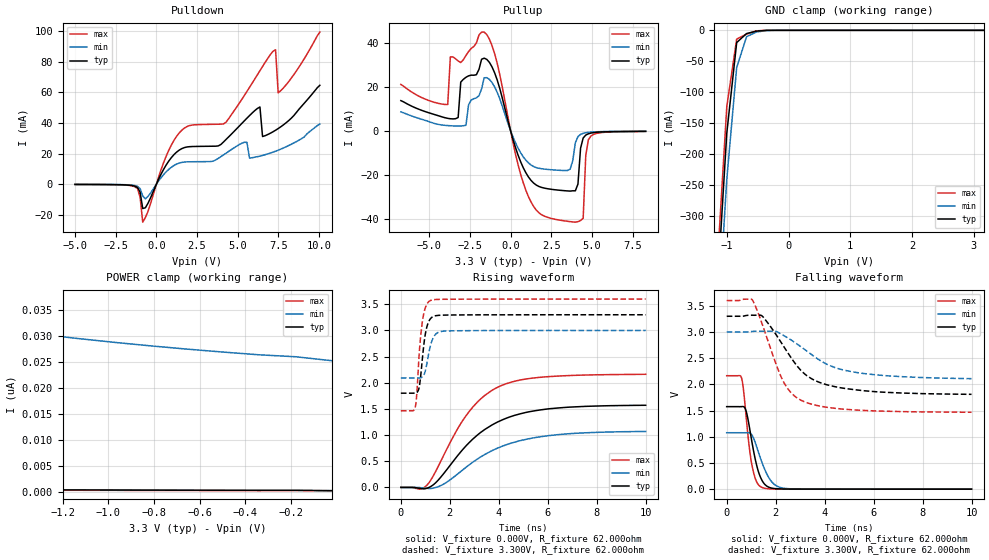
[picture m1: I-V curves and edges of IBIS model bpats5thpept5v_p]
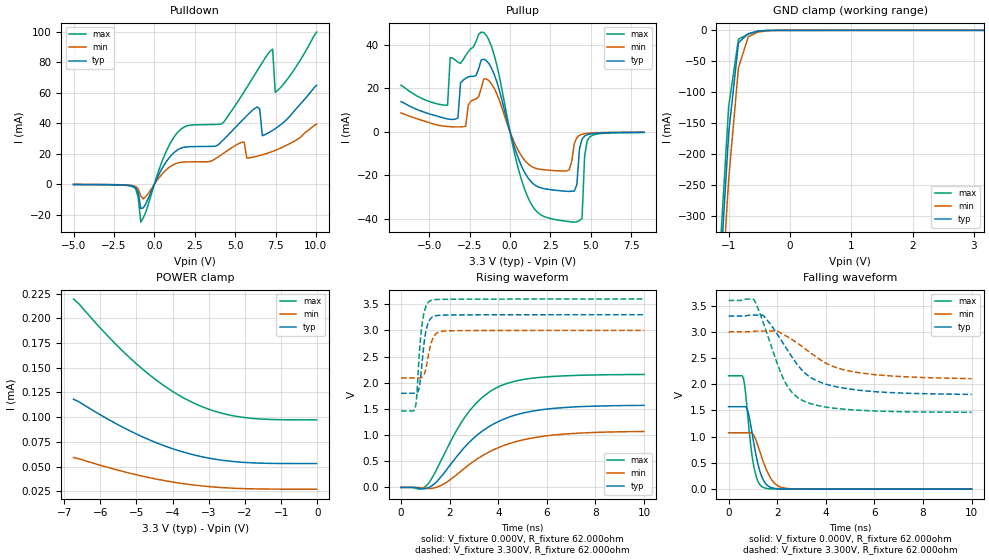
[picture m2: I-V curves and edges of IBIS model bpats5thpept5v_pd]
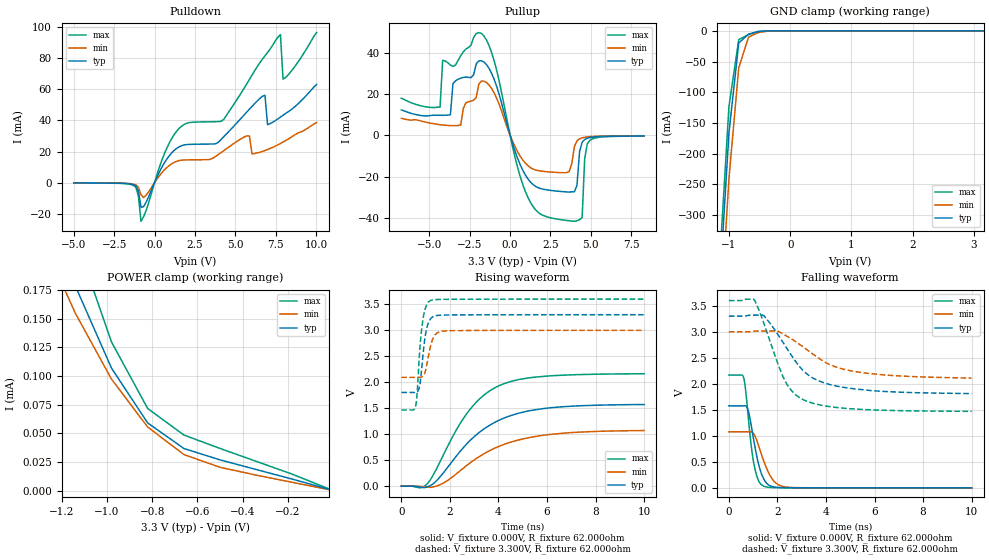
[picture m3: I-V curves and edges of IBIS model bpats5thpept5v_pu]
[IBIS Ver]  4.0
[File Name]  lpc13xx_hvqfn33_rev.ibs
[File Rev]  1.0
[Date]   Fri Oct 15 17:01:21 PDT 2006
[Source]   Package model from Ansoft Q3D Extractor 7.1.1
[Notes]   IO models Rev 0.20 IBIS Model Design Automation Generation
[Copyright] NXP Semiconductors 2006. All rights reserved.
|   LPC134x/LPC131x IBIS Model
[Disclaimer]
| NXP Semiconductors warrants and represents that the IBIS models
| identified herein are owned by NXP Semiconductors (NXP).  The
| models provided are not warranted as fully representing all of the
| operating characteristics and specifications of the semiconductor
| products to which the models relate.  Moreover, unless there is a
| signed, written agreement to the contrary, these models are furnished
| on an "as is" basis without support or warranty of any kind, either
| expressed or implied, regarding the use thereof, and NXP
| specifically disclaims all implied warranties of merchantability and
| fitness of the models for any purpose.
| NXP does not assume any liability arising out of the application
| or use of these IBIS models including infringement of patents and
| copyrights, nor does NXP convey any license under its patents and
| copyrights or the rights of others.
| NXP provides IBIS models as a service to our customers.  You and
| your company shall not distribute, convey, sell, or give these models
| to anyone else without receiving prior written permission from
| NXP.
[Component]   lpc13xx
[Manufacturer]  NXP
[Package]
|   Typ   Min   Max
R_pkg   1.15e-1   0.24e-1   4.46e-1
L_pkg   6.44e-9   5.71e-9   7.17e-9
C_pkg   0.5e-12   0.5e-12   0.5e-12
| (Pin and IO model definitions)
| IMPORTANT NOTES:
| The lpc13xx GPIO pins, excluding the I2C, have programmable input
| configurations. For this reason, three models are supplied for those basic
| padcells. Each model is identified by a unique suffix code at the end of
| the modelname:
| _p=plain input, _pd=pulldown enabled, _pu=pullup enabled
| The model_name for each of the GPIO pins in the [Pin] table below reflects
| the default state of that pin on power up (input with pullup enabled).
| The user may modify the model_name for a specific P#.# pin if that pin's
| input configuration is programmed differently from the default in the
| actual application. However, the model_names for all other pins are
| non-configurable and should not be altered.
| All GPIO padcells have 5ns slew rate control when operated as outputs,
| unless otherwise noted.
|This model covers both the USB version LPC134x and the non usb version
|of the LPC1300. Uncomment the appropriate model for the correct function.
[Pin]   signal_name   model_name   | comments
1   PIO2_0   bpts5ptpht5v_pu
2   PIO0_0   bpts5ptpht5v_pu   | Reset Pad
3   PIO0_1   bpts5ptpht5v_pu
4   XTALIN   NC
5   XTALOUT   NC
6   VDDIO_EXT_1   POWER
7   PIO1_8   bpts5ptpht5v_pu
8   PIO0_2   bpts5ptpht5v_pu
9   PIO0_3   bpts5ptpht5v_pu
10   PIO0_4   iic3m4sdat5v_400k   |iic3m20m4sdat5v_pd
11   PIO0_5   iic3m4sdat5v_400k   |iic3m20m4sdat5v_pd
12   PIO1_9   bpts5ptpht5v_pu
13   USB_DM   usb11f1_iom_hs
14   USB+DP   usb11f1_iop_hs
|13   PIO3_4   bpts5ptpht5v_pu
|14   PIO3_5   bpts5ptpht5v_pu
15   PIO0_6   bpts5ptpht5v_pu
16   PIO0_7   bpts5ptpht5v_pu   |bpt20ms5ptpht5v_pd_v1
17   PIO0_8   bpts5ptpht5v_pu
18   PIO0_9   bpts5ptpht5v_pu
19   PIO0_10   bpts5ptpht5v_pu
20   PIO1_10   bpats5thpept5v_pu
21   PIO0_11   bpats5thpept5v_pu
22   PIO1_0   bpats5thpept5v_pu
23   PIO1_1   bpats5thpept5v_pu
24   PIO1_2   bpats5thpept5v_pu
25   PIO1_3   bpats5thpept5v_pu
26   PIO1_4   bpats5thpept5v_pu   |bpats5thpept5v_pdwu_v1
27   PIO1_11   bpats5thpept5v_pu
28   PIO3_2   bpts5ptpht5v_pu
29   VDDMAIN_EXT   POWER
30   PIO1_5   bpts5ptpht5v_pu
31   PIO1_6   bpts5ptpht5v_pu
32   PIO1_7   bpts5ptpht5v_pu
| Models and submodels in the file (9): bpats5thpept5v_p (I/O), bpats5thpept5v_pd (I/O), bpats5thpept5v_pu (I/O), bpts5ptpht5v_p (I/O), bpts5ptpht5v_pd (I/O), bpts5ptpht5v_pu (I/O), iic3m4sdat5v_400k (I/O_open_drain), usb11f1_iom_hs (I/O), usb11f1_iop_hs (I/O)
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| bpats5thpept5v
|   Bidirectional Pad 3v3
|   CMOS
|   Characterized at Core 1.8V and I/O 3.3V
| Plain input Mode (p1=0, p2=1)
[Model]   bpats5thpept5v_p | of bpats5thpept5v
Model_type   I/O
Polarity   Non-Inverting
Enable   Active-Low
|  Reciever Thresholds
Vinl   = 0.54V
Vinh   = 1.26V
| AC Test Load Conditions
Vref   = 0
Cref   = 1.2e-11
Rref   = 1000000000
Vmeas   = 0.9
| [Process Range]   typical   min   max
| C_comp edge width   400.000ps   400.000ps   400.000ps
| C_comp Tstrobe   40.000fs   40.000fs   40.000fs
C_comp   2.539pF   2.402pF   2.679pF
[Temperature Range]   25   125   -40
[Voltage Range]   3.30V   3.00V   3.60V
[GND Clamp Reference]   0.00V   0.00V   0.00V
[Pulldown Reference]   0.00V   0.00V   0.00V
[POWER Clamp Reference]   3.30V   3.00V   3.60V
[Pullup Reference]   3.30V   3.00V   3.60V
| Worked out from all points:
|   slope of the pulldown table from 0 to 0.495 V, typ, clamps not added: 46.5 ohm
|   slope of the pullup table from 0 to 0.495 V, typ, clamps not added: 41.9 ohm
|   GND clamp passes 1 mA (typ) near -0.48 V on its own axis
|   rising waveform, V_fixture 0.000V, R_fixture 62.000ohm: 20-80 % time 2.15ns typ, 2.37ns min, 1.8ns max; typ from 0 V to 1.57 V
|   falling waveform, V_fixture 0.000V, R_fixture 62.000ohm: 20-80 % time 411ps typ, 539ps min, 319ps max; typ from 1.57 V to 0 V
|   rising waveform, V_fixture 3.300V, R_fixture 62.000ohm: 20-80 % time 225ps typ, 260ps min, 215ps max; typ from 1.8 V to 3.3 V
|   falling waveform, V_fixture 3.300V, R_fixture 62.000ohm: 20-80 % time 1.53ns typ, 1.95ns min, 1.1ns max; typ from 3.3 V to 1.81 V
[GND Clamp]
| ref voltage   0.00V   0.00V   0.00V
|   Voltage   I(typ)   I(min)   I(max)
-5V       -7.933A    -7.953A    -7.929A
-1.16V    -429.6mA   -501mA     -389.4mA
-1V       -166.1mA   -240.8mA   -123.1mA
-840mV    -19.82mA   -60.19mA   -14.18mA
-680mV    -5.225mA   -10.28mA   -6.152mA
-520mV    -1.304mA   -2.7mA     -818.1uA
-200mV    -132.3nA   -9.731uA   -2.769nA
3.16V     216.3pA    26.32nA    148.8pA
[Power Clamp]   | Vtable = Vcc - Vpad
| ref voltage   3.30V   3.00V   3.60V
|   Voltage   I(typ)   I(min)   I(max)
-6.74V    1.379nA    125.5nA    723.8pA
-4.66V    863pA      70.57nA    560.5pA
-2.42V    509.5pA    38.28nA    388.3pA
-2.26V    489.9pA    36.89nA    376pA
-2.1V     470.8pA    35.59nA    363.8pA
-1.78V    434.1pA    33.27nA    339.4pA
-1.62V    416.5pA    32.24nA    327.2pA
-1.3V     382.5pA    30.41nA    302.8pA
-820mV    334.3pA    28.18nA    266.3pA
-340mV    288.9pA    26.43nA    229.9pA
-180mV    281.7pA    26.06nA    265.9pA
-20mV     233pA      25.29nA    176.8pA
[Pulldown]
| ref voltage   0.00V   0.00V   0.00V
|   Voltage   I(typ)   I(min)   I(max)
-5V       -187.5uA   -145.8uA   -211.8uA
-1.32V    -1.32mA    -939.5uA   -1.723mA
-1V       -5.324mA   -2.961mA   -8.618mA
-840mV    -15.95mA   -7.735mA   -24.89mA
1.4V      22.26mA    13.79mA    33.48mA
4.28V     29.27mA    20.27mA    40.55mA
5.56V     43.15mA    27.33mA    60.63mA
6.36V     50.49mA    18.36mA    74.24mA
6.52V     31.16mA    18.79mA    76.97mA
7.32V     35.27mA    21.55mA    87.95mA
7.48V     36.36mA    22.22mA    59.78mA
10.04V    64.68mA    39.32mA    99.49mA
[Pullup]   | Vtable = Vcc - Vpad
| ref voltage   3.30V   3.00V   3.60V
|   Voltage   I(typ)   I(min)   I(max)
-6.74V    13.67mA    8.53mA     21.02mA
-3.86V    5.598mA    2.307mA    11.88mA
-3.7V     5.416mA    2.227mA    33.56mA
-2.74V    24.29mA    2.441mA    34.22mA
-1.62V    32.99mA    24.07mA    44.83mA
940mV     -19.18mA   -13.46mA   -27.14mA
2.86V     -27.01mA   -17.98mA   -40.52mA
3.98V     -27.37mA   -5.511mA   -41.66mA
4.46V     -3.36mA    -1.235mA   -39.89mA
4.62V     -2.02mA    -961.6uA   -11.27mA
4.94V     -1.105mA   -662.3uA   -2.417mA
8.3V      -310.5uA   -276.1uA   -365.1uA
[Ramp]
R_load   = 62.000ohm
|   dV/dt(typ)   dV/dt(min)   dV/dt(max)
dV/dt_r   720.631mV/2.205ns   482.682mV/2.365ns   1.049V/2.035ns
dV/dt_f   674.653mV/1.565ns   397.637mV/1.940ns   1.038V/1.245ns
[Rising Waveform]  | cubic spline decimation from 2001 points
V_fixture   = 0.000V
R_fixture   = 62.000ohm
|   Time   V(typ)   V(min)   V(max)
0s        2.482nV    412.2nV    1.344nV
765ps     -17.12mV   -3.168mV   -33.52mV
1.06ns    -16.23mV   -17.53mV   40.55mV
1.715ns   244.2mV    54.65mV    580.5mV
2.665ns   795.4mV    385.7mV    1.372V
3.255ns   1.049V     581mV      1.689V
3.95ns    1.25V      750.6mV    1.914V
4.895ns   1.409V     895.8mV    2.055V
6.08ns    1.504V     991.8mV    2.119V
10ns      1.57V      1.07V      2.162V
[Falling Waveform]  | cubic spline decimation from 2001 points
V_fixture   = 0.000V
R_fixture   = 62.000ohm
|   Time   V(typ)   V(min)   V(max)
0s        1.575V     1.077V     2.165V
610ps     1.576V     1.077V     2.118V
680ps     1.576V     1.076V     1.921V
790ps     1.496V     1.077V     1.406V
1.025ns   917.9mV    1.038V     476.3mV
1.205ns   493mV      837.1mV    157.9mV
1.445ns   165.7mV    505.2mV    32.07mV
1.885ns   16.15mV    117.4mV    4.029mV
2.4ns     2.893mV    14.38mV    1.574mV
10ns      49.83uV    118.5uV    23.14uV
[Rising Waveform]  | cubic spline decimation from 2001 points
V_fixture   = 3.300V
V_fixture_min = 3.000V
V_fixture_max = 3.600V
R_fixture   = 62.000ohm
|   Time   V(typ)   V(min)   V(max)
0s        1.801V     2.092V     1.464V
585ps     1.801V     2.093V     1.532V
640ps     1.809V     2.093V     1.718V
755ps     1.929V     2.092V     2.589V
885ps     2.487V     2.116V     3.188V
1.03ns    3.005V     2.289V     3.47V
1.21ns    3.225V     2.71V      3.572V
1.41ns    3.281V     2.923V     3.591V
1.82ns    3.294V     2.989V     3.596V
10ns      3.3V       3V         3.6V
[Falling Waveform]  | cubic spline decimation from 2001 points
V_fixture   = 3.300V
V_fixture_min = 3.000V
V_fixture_max = 3.600V
R_fixture   = 62.000ohm
|   Time   V(typ)   V(min)   V(max)
0s        3.3V       3V         3.6V
1.04ns    3.32V      3.009V     3.616V
1.45ns    3.304V     3.014V     3.151V
2.045ns   2.929V     3.004V     2.35V
2.325ns   2.727V     2.933V     2.045V
2.66ns    2.488V     2.839V     1.826V
3.1ns     2.235V     2.695V     1.683V
4.145ns   1.986V     2.371V     1.559V
5.13ns    1.904V     2.24V      1.515V
10ns      1.81V      2.109V     1.468V
| bpats5thpept5v
|   Bidirectional Pad 3v3
|   CMOS
|   Characterized at Core 1.8V and I/O 3.3V
| Pull Down Mode (p1=1, p2=1)
[Model]   bpats5thpept5v_pd | of bpats5thpept5v
Model_type   I/O
Polarity   Non-Inverting
Enable   Active-Low
|  Reciever Thresholds
Vinl   = 0.54V
Vinh   = 1.26V
| AC Test Load Conditions
Vref   = 0
Cref   = 1.2e-11
Rref   = 1000000000
Vmeas   = 0.9
| [Process Range]   typical   min   max
| C_comp edge width   400.000ps   400.000ps   400.000ps
| C_comp Tstrobe   40.000fs   40.000fs   40.000fs
C_comp   2.538pF   2.399pF   2.678pF
[Temperature Range]   25   125   -40
[Voltage Range]   3.30V   3.00V   3.60V
[GND Clamp Reference]   0.00V   0.00V   0.00V
[Pulldown Reference]   0.00V   0.00V   0.00V
[POWER Clamp Reference]   3.30V   3.00V   3.60V
[Pullup Reference]   3.30V   3.00V   3.60V
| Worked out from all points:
|   slope of the pulldown table from 0 to 0.495 V, typ, clamps not added: 46.5 ohm
|   slope of the pullup table from 0 to 0.495 V, typ, clamps not added: 41.9 ohm
|   GND clamp passes 1 mA (typ) near -0.48 V on its own axis
|   rising waveform, V_fixture 0.000V, R_fixture 62.000ohm: 20-80 % time 2.15ns typ, 2.37ns min, 1.8ns max; typ from 0 V to 1.57 V
|   falling waveform, V_fixture 0.000V, R_fixture 62.000ohm: 20-80 % time 410ps typ, 538ps min, 318ps max; typ from 1.57 V to 0 V
|   rising waveform, V_fixture 3.300V, R_fixture 62.000ohm: 20-80 % time 227ps typ, 261ps min, 216ps max; typ from 1.8 V to 3.3 V
|   falling waveform, V_fixture 3.300V, R_fixture 62.000ohm: 20-80 % time 1.53ns typ, 1.95ns min, 1.1ns max; typ from 3.3 V to 1.81 V
[GND Clamp]
| ref voltage   0.00V   0.00V   0.00V
|   Voltage   I(typ)   I(min)   I(max)
-5V       -7.933A    -7.953A    -7.929A
-1.16V    -429.6mA   -501mA     -389.4mA
-1V       -166.1mA   -240.8mA   -123.1mA
-840mV    -19.84mA   -60.2mA    -14.2mA
-680mV    -5.244mA   -10.3mA    -6.181mA
-520mV    -1.329mA   -2.711mA   -860.7uA
-200mV    -17.4uA    -20.02uA   -26.89uA
3.16V     53.01uA    27.08uA    97.28uA
[Power Clamp]   | Vtable = Vcc - Vpad
| ref voltage   3.30V   3.00V   3.60V
|   Voltage   I(typ)   I(min)   I(max)
-6.74V    118.1uA    59.14uA    219.6uA
-6.58V    115.3uA    57.74uA    214.3uA
-6.1V     104.5uA    52.36uA    194.3uA
-5.62V    94.49uA    47.37uA    175.6uA
-4.98V    82.54uA    41.46uA    153.3uA
-4.5V     74.82uA    37.65uA    138.8uA
-4.18V    70.31uA    35.43uA    130.3uA
-3.54V    62.97uA    31.84uA    116.5uA
-2.9V     57.87uA    29.37uA    106.8uA
-2.1V     54.38uA    27.71uA    100uA
-1.3V     53.2uA     27.16uA    97.67uA
-20mV     53.01uA    27.08uA    97.29uA
[Pulldown]
| ref voltage   0.00V   0.00V   0.00V
|   Voltage   I(typ)   I(min)   I(max)
-5V       -187.5uA   -145.8uA   -211.8uA
-1.32V    -1.32mA    -939.5uA   -1.723mA
-1V       -5.324mA   -2.961mA   -8.619mA
-840mV    -15.95mA   -7.735mA   -24.89mA
1.4V      22.26mA    13.79mA    33.48mA
4.28V     29.29mA    20.29mA    40.56mA
5.56V     43.21mA    27.5mA     60.72mA
6.36V     50.67mA    18.36mA    74.36mA
6.68V     31.78mA    19.27mA    79.81mA
7.32V     35.33mA    21.55mA    88.56mA
7.48V     36.44mA    22.22mA    60.22mA
10.04V    64.83mA    39.4mA     99.75mA
[Pullup]   | Vtable = Vcc - Vpad
| ref voltage   3.30V   3.00V   3.60V
|   Voltage   I(typ)   I(min)   I(max)
-6.74V    13.82mA    8.599mA    21.35mA
-3.86V    5.864mA    2.372mA    12.19mA
-3.7V     5.685mA    2.288mA    34.11mA
-2.74V    24.57mA    2.531mA    35.04mA
-1.62V    33.35mA    24.26mA    45.59mA
940mV     -19.18mA   -13.46mA   -27.15mA
2.86V     -27.01mA   -17.98mA   -40.52mA
3.98V     -27.37mA   -5.511mA   -41.66mA
4.46V     -3.361mA   -1.235mA   -39.89mA
4.62V     -2.02mA    -961.6uA   -11.27mA
4.94V     -1.105mA   -662.3uA   -2.418mA
8.3V      -310.5uA   -276.1uA   -365.1uA
[Ramp]
R_load   = 62.000ohm
|   dV/dt(typ)   dV/dt(min)   dV/dt(max)
dV/dt_r   719.302mV/2.205ns   482.029mV/2.365ns   1.047V/2.040ns
dV/dt_f   675.416mV/1.570ns   397.994mV/1.940ns   1.039V/1.245ns
[Rising Waveform]  | cubic spline decimation from 2001 points
V_fixture   = 0.000V
R_fixture   = 62.000ohm
|   Time   V(typ)   V(min)   V(max)
0s        2.445nV    410.1nV    1.304nV
765ps     -17.11mV   -3.168mV   -33.47mV
1.06ns    -16.17mV   -17.52mV   40.67mV
1.685ns   226.6mV    47.31mV    550.5mV
2.675ns   798.3mV    388.8mV    1.374V
3.335ns   1.074V     602.8mV    1.717V
4.07ns    1.273V     772.5mV    1.936V
4.98ns    1.416V     903.8mV    2.058V
6.15ns    1.504V     994mV      2.117V
10ns      1.567V     1.068V     2.158V
[Falling Waveform]  | cubic spline decimation from 2001 points
V_fixture   = 0.000V
R_fixture   = 62.000ohm
|   Time   V(typ)   V(min)   V(max)
0s        1.572V     1.075V     2.162V
610ps     1.573V     1.075V     2.114V
680ps     1.573V     1.075V     1.917V
790ps     1.493V     1.076V     1.401V
1.025ns   915mV      1.036V     471.2mV
1.195ns   510.1mV    849.5mV    165.8mV
1.415ns   190.6mV    541.8mV    37.07mV
1.875ns   16.42mV    121.2mV    3.959mV
2.38ns    2.935mV    15.21mV    1.58mV
10ns      49.48uV    118uV      22.85uV
[Rising Waveform]  | cubic spline decimation from 2001 points
V_fixture   = 3.300V
V_fixture_min = 3.000V
V_fixture_max = 3.600V
R_fixture   = 62.000ohm
|   Time   V(typ)   V(min)   V(max)
0s        1.798V     2.091V     1.461V
590ps     1.799V     2.091V     1.537V
640ps     1.806V     2.091V     1.714V
755ps     1.926V     2.091V     2.583V
875ps     2.436V     2.11V      3.148V
1.015ns   2.967V     2.256V     3.446V
1.21ns    3.222V     2.708V     3.568V
1.415ns   3.279V     2.923V     3.588V
1.79ns    3.292V     2.987V     3.593V
10ns      3.299V     2.999V     3.598V
[Falling Waveform]  | cubic spline decimation from 2001 points
V_fixture   = 3.300V
V_fixture_min = 3.000V
V_fixture_max = 3.600V
R_fixture   = 62.000ohm
|   Time   V(typ)   V(min)   V(max)
0s        3.299V     2.999V     3.598V
1.035ns   3.318V     3.008V     3.614V
1.45ns    3.301V     3.013V     3.145V
2.005ns   2.954V     3.008V     2.395V
2.305ns   2.738V     2.937V     2.059V
2.63ns    2.506V     2.846V     1.835V
3.07ns    2.245V     2.704V     1.685V
4.13ns    1.985V     2.373V     1.556V
5.155ns   1.899V     2.236V     1.51V
10ns      1.807V     2.107V     1.465V
| bpats5thpept5v
|   Bidirectional Pad 3v3
|   CMOS
|   Characterized at Core 1.8V and I/O 3.3V
| Pull Up Mode (p1=0, p2=0)
[Model]   bpats5thpept5v_pu | of bpats5thpept5v
Model_type   I/O
Polarity   Non-Inverting
Enable   Active-Low
|  Reciever Thresholds
Vinl   = 0.54V
Vinh   = 1.26V
| AC Test Load Conditions
Vref   = 0
Cref   = 1.2e-11
Rref   = 1000000000
Vmeas   = 0.9
| [Process Range]   typical   min   max
| C_comp edge width   400.000ps   400.000ps   400.000ps
| C_comp Tstrobe   40.000fs   40.000fs   40.000fs
C_comp   2.536pF   2.398pF   2.677pF
[Temperature Range]   25   125   -40
[Voltage Range]   3.30V   3.00V   3.60V
[GND Clamp Reference]   0.00V   0.00V   0.00V
[Pulldown Reference]   0.00V   0.00V   0.00V
[POWER Clamp Reference]   3.30V   3.00V   3.60V
[Pullup Reference]   3.30V   3.00V   3.60V
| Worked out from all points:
|   slope of the pulldown table from 0 to 0.495 V, typ, clamps not added: 46.5 ohm
|   slope of the pullup table from 0 to 0.495 V, typ, clamps not added: 41.9 ohm
|   GND clamp passes 1 mA (typ) near -0.48 V on its own axis
|   POWER clamp passes 1 mA (typ) near -2.29 V on its own axis
|   rising waveform, V_fixture 0.000V, R_fixture 62.000ohm: 20-80 % time 2.14ns typ, 2.37ns min, 1.8ns max; typ from 0.001 V to 1.57 V
|   falling waveform, V_fixture 0.000V, R_fixture 62.000ohm: 20-80 % time 411ps typ, 539ps min, 320ps max; typ from 1.58 V to 0.001 V
|   rising waveform, V_fixture 3.300V, R_fixture 62.000ohm: 20-80 % time 224ps typ, 260ps min, 214ps max; typ from 1.8 V to 3.3 V
|   falling waveform, V_fixture 3.300V, R_fixture 62.000ohm: 20-80 % time 1.53ns typ, 1.95ns min, 1.1ns max; typ from 3.3 V to 1.81 V
[GND Clamp]
| ref voltage   0.00V   0.00V   0.00V
|   Voltage   I(typ)   I(min)   I(max)
-5V       -7.933A    -7.953A    -7.929A
-1.16V    -429.6mA   -501mA     -389.4mA
-1V       -166.1mA   -240.8mA   -123.1mA
-840mV    -19.83mA   -60.19mA   -14.19mA
-680mV    -5.242mA   -10.3mA    -6.178mA
-520mV    -1.331mA   -2.714mA   -864.2uA
-200mV    -50.25uA   -41.81uA   -77.56uA
3.16V     -7.353uA   6.327uA    -29.63uA
[Power Clamp]   | Vtable = Vcc - Vpad
| ref voltage   3.30V   3.00V   3.60V
|   Voltage   I(typ)   I(min)   I(max)
-6.74V    8.239mA    4.142mA    14.64mA
-1.3V     267.9uA    224.8uA    334.3uA
-1.14V    178.7uA    154.9uA    220.9uA
-980mV    106.8uA    97.21uA    129.7uA
-820mV    58.96uA    55.39uA    71.57uA
-660mV    36.65uA    31.38uA    48.44uA
-500mV    26.73uA    20.24uA    36.7uA
-180mV    9.891uA    7.111uA    14.19uA
-20mV     1.102uA    817.7nA    1.531uA
[Pulldown]
| ref voltage   0.00V   0.00V   0.00V
|   Voltage   I(typ)   I(min)   I(max)
-5V       -187.5uA   -145.8uA   -211.8uA
-1.32V    -1.32mA    -939.5uA   -1.723mA
-840mV    -15.95mA   -7.735mA   -24.89mA
1.56V     23.24mA    14.25mA    35.29mA
4.28V     29.46mA    20.48mA    40.61mA
5.72V     45.48mA    30.13mA    63.63mA
6.84V     56.23mA    20.64mA    81.58mA
7V        37.28mA    21.27mA    83.66mA
7.8V      42.14mA    25.2mA     95.19mA
7.96V     43.32mA    26.11mA    66.52mA
8.12V     44.49mA    27.07mA    67.59mA
10.04V    63.09mA    38.66mA    96.53mA
[Pullup]   | Vtable = Vcc - Vpad
| ref voltage   3.30V   3.00V   3.60V
|   Voltage   I(typ)   I(min)   I(max)
-6.74V    12.27mA    8.208mA    17.93mA
-4.34V    9.688mA    5.132mA    13.69mA
-4.18V    9.676mA    4.983mA    36.31mA
-3.06V    27.66mA    4.956mA    38.56mA
-1.78V    36.09mA    26.29mA    49.34mA
940mV     -19.18mA   -13.46mA   -27.14mA
3.02V     -27.13mA   -18.05mA   -40.73mA
3.98V     -27.37mA   -5.511mA   -41.66mA
4.46V     -3.361mA   -1.235mA   -39.89mA
4.62V     -2.02mA    -961.6uA   -11.27mA
4.94V     -1.105mA   -662.3uA   -2.418mA
8.3V      -310.5uA   -276.1uA   -365.1uA
[Ramp]
R_load   = 62.000ohm
|   dV/dt(typ)   dV/dt(min)   dV/dt(max)
dV/dt_r   721.276mV/2.205ns   483.044mV/2.365ns   1.050V/2.040ns
dV/dt_f   673.548mV/1.570ns   397.074mV/1.940ns   1.036V/1.245ns
[Rising Waveform]  | cubic spline decimation from 2001 points
V_fixture   = 0.000V
R_fixture   = 62.000ohm
|   Time   V(typ)   V(min)   V(max)
0s        1.219mV    1.008mV    1.479mV
765ps     -15.82mV   -2.159mV   -31.04mV
1.06ns    -13.88mV   -16.43mV   44.85mV
1.715ns   248mV      56.81mV    587.1mV
2.695ns   814.7mV    399.6mV    1.397V
3.235ns   1.045V     578mV      1.685V
3.985ns   1.261V     760.1mV    1.926V
4.8ns     1.401V     886.9mV    2.049V
5.97ns    1.501V     987.6mV    2.118V
10ns      1.572V     1.072V     2.164V
[Falling Waveform]  | cubic spline decimation from 2001 points
V_fixture   = 0.000V
R_fixture   = 62.000ohm
|   Time   V(typ)   V(min)   V(max)
0s        1.577V     1.078V     2.168V
605ps     1.578V     1.078V     2.128V
680ps     1.578V     1.078V     1.924V
790ps     1.499V     1.079V     1.41V
1.025ns   920.6mV    1.039V     480.1mV
1.21ns    485.9mV    831.8mV    153mV
1.415ns   193.6mV    545.1mV    38.94mV
1.845ns   19.81mV    137.4mV    6.125mV
2.33ns    4.655mV    18.77mV    3.371mV
10ns      1.272mV    1.133mV    1.504mV
[Rising Waveform]  | cubic spline decimation from 2001 points
V_fixture   = 3.300V
V_fixture_min = 3.000V
V_fixture_max = 3.600V
R_fixture   = 62.000ohm
|   Time   V(typ)   V(min)   V(max)
0s        1.804V     2.094V     1.467V
585ps     1.804V     2.094V     1.535V
640ps     1.811V     2.094V     1.722V
745ps     1.908V     2.094V     2.524V
880ps     2.466V     2.115V     3.176V
1.01ns    2.96V      2.249V     3.45V
1.2ns     3.219V     2.693V     3.573V
1.425ns   3.282V     2.93V      3.592V
1.755ns   3.293V     2.987V     3.596V
10ns      3.3V       3V         3.6V
[Falling Waveform]  | cubic spline decimation from 2001 points
V_fixture   = 3.300V
V_fixture_min = 3.000V
V_fixture_max = 3.600V
R_fixture   = 62.000ohm
|   Time   V(typ)   V(min)   V(max)
0s        3.3V       3V         3.6V
1.04ns    3.32V      3.009V     3.616V
1.45ns    3.304V     3.014V     3.152V
2.045ns   2.93V      3.004V     2.354V
2.325ns   2.728V     2.933V     2.048V
2.68ns    2.477V     2.833V     1.821V
3.07ns    2.251V     2.706V     1.693V
3.76ns    2.046V     2.474V     1.593V
4.99ns    1.914V     2.253V     1.522V
10ns      1.812V     2.11V      1.471V
